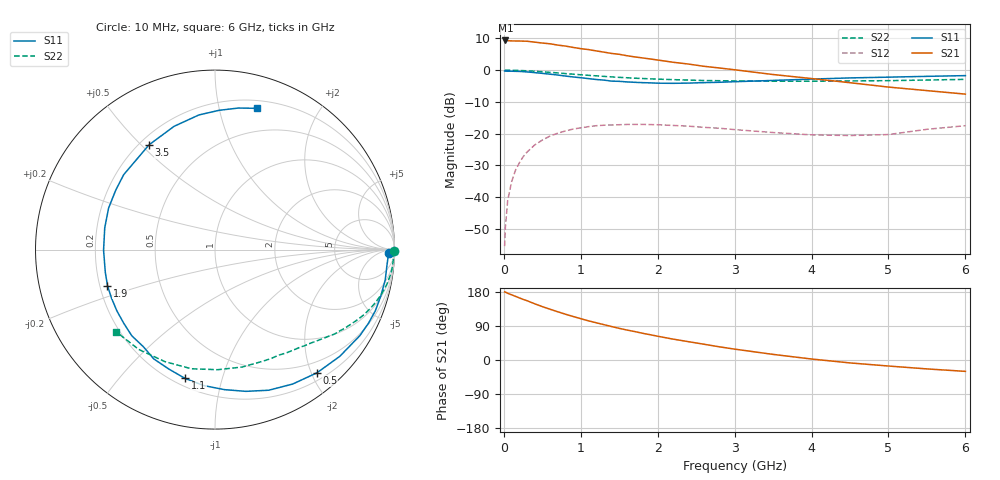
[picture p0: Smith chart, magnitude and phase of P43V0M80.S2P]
! SIEMENS Small Signal Semiconductors
! BFP182
! Si NPN RF Bipolar Junction Transistor in SOT143
! VCE = 3 V  IC = 0.8 mA
! Common Emitter S-Parameters:  March  1996
# GHz  S  MA  R  50
!  f  S11  S21  S12  S22
! GHz  MAG  ANG  MAG  ANG  MAG  ANG  MAG  ANG
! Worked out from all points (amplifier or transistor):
!   36 points, 10 MHz to 6 GHz, reference 50 ohm
!   highest |S21| = 9.4 dB at 20 MHz (marker M1)
!   |S21| within 3 dB of that: start of sweep to 1.131 GHz
!   unconditionally stable (mu >= 1): 2.759 GHz to end of sweep
!   at 250 MHz: K = 0.09, MSG = 18.2 dB, |S12| = -27.3 dB
!   at 1.4 GHz: K = 0.52, MSG = 11.3 dB, |S12| = -17.2 dB
!   at 6 GHz: K = 1.08, MAG = 3.2 dB, |S12| = -17.5 dB
!   S11 on the Smith chart (normalised r, x): 10 MHz: 50, -29; 500 MHz: 0.31, -2.09; 1.1 GHz: 0.24, -0.76; 1.9 GHz: 0.23, -0.15; 3.5 GHz: 0.24, +0.53; 6 GHz: 0.27, +1.30
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0.01  0.9707 -1.0  2.903 179.6  0.0017 84.3  0.9982 -0.4
0.02  0.966 -2.0  2.935 179.1  0.0034 88.7  0.9983 -0.8
0.05  0.962 -5.3  2.91 176.1  0.0089 88.6  0.9978 -1.9
0.1  0.9634 -10.1  2.889 172.1  0.0174 82.4  0.9943 -3.8
0.15  0.9592 -15.7  2.88 168.1  0.0264 79.8  0.993 -5.7
0.3  0.9389 -30.7  2.854 156.6  0.0512 71.1  0.9777 -11.2
0.4  0.915 -40.5  2.762 148.4  0.0664 64.5  0.9621 -14.6
0.5  0.8911 -50.4  2.672 140.9  0.0794 58.4  0.9444 -17.8
0.6  0.865 -60.0  2.602 134.0  0.0919 52.9  0.9245 -20.9
0.8  0.8083 -77.7  2.395 120.9  0.1105 42.6  0.8839 -26.3
1.1  0.7367 -103.1  2.109 103.3  0.1292 30.1  0.8296 -33.1
1.3  0.6982 -119.2  1.923 93.3  0.136 22.7  0.7987 -37.0
1.5  0.6674 -134.0  1.776 83.5  0.1385 16.7  0.7705 -40.6
1.9  0.6317 -161.5  1.502 66.8  0.1393 6.6  0.7314 -47.2
2.2  0.6209 -179.7  1.332 55.1  0.135 1.2  0.7098 -52.1
2.8  0.6447 149.0  1.083 34.8  0.122 -6.4  0.6827 -62.6
3.5  0.6897 122.2  0.854 14.8  0.1044 -7.9  0.6716 -76.9
4  0.7236 108.4  0.738 2.6  0.0959 -3.2  0.6693 -88.6
4.5  0.7556 96.8  0.635 -7.7  0.0937 2.6  0.6769 -101.2
5  0.7764 88.3  0.542 -15.9  0.097 12.9  0.6838 -114.1
5.5  0.7995 80.6  0.477 -23.5  0.1173 15.9  0.6999 -127.4
6  0.8208 73.5  0.42 -30.0  0.1337 15.2  0.7165 -140.3
